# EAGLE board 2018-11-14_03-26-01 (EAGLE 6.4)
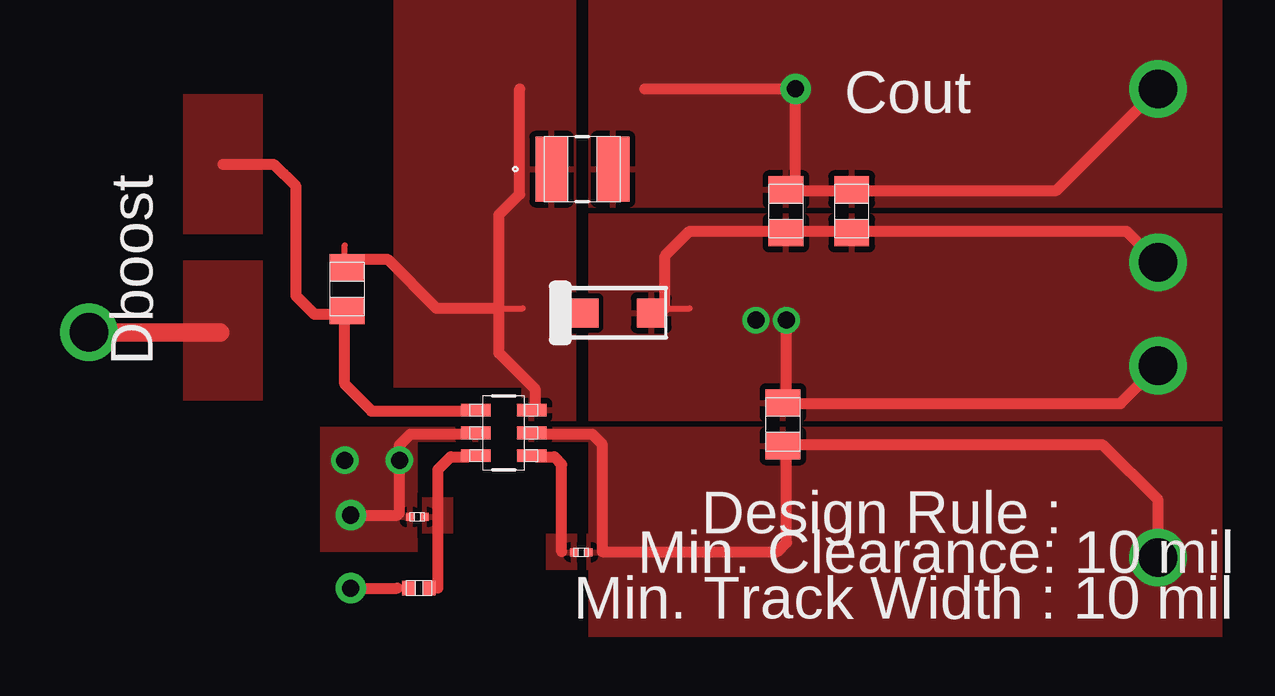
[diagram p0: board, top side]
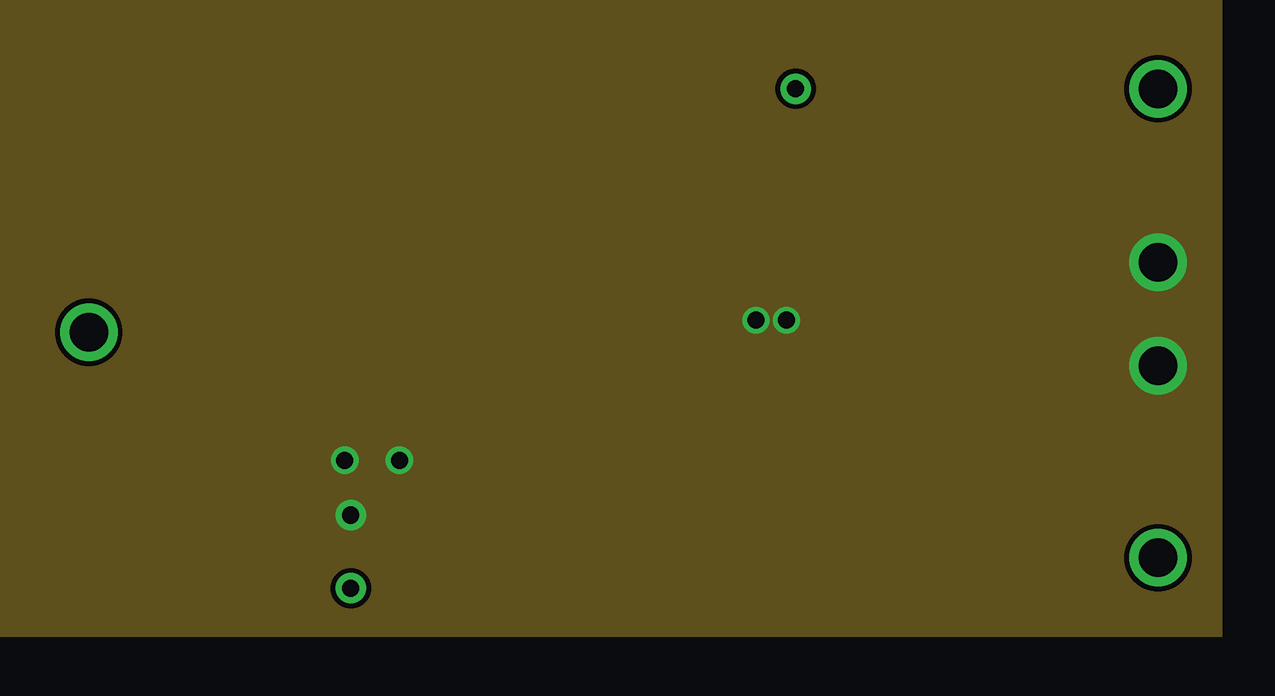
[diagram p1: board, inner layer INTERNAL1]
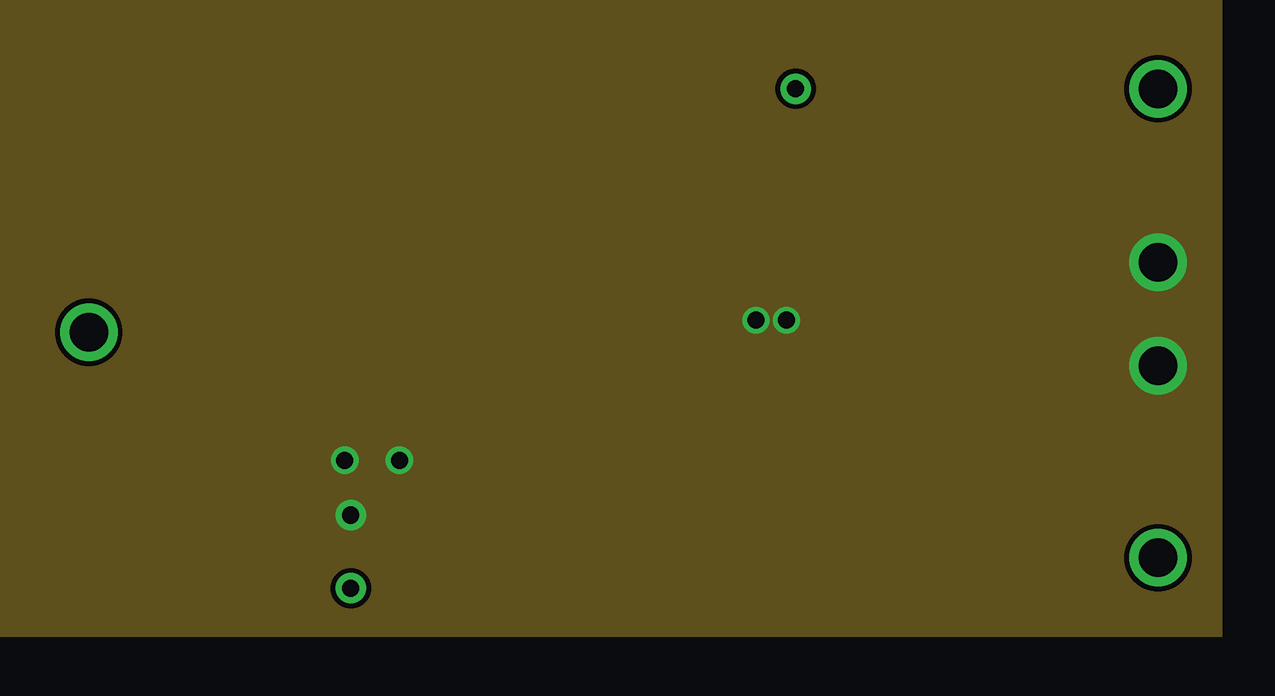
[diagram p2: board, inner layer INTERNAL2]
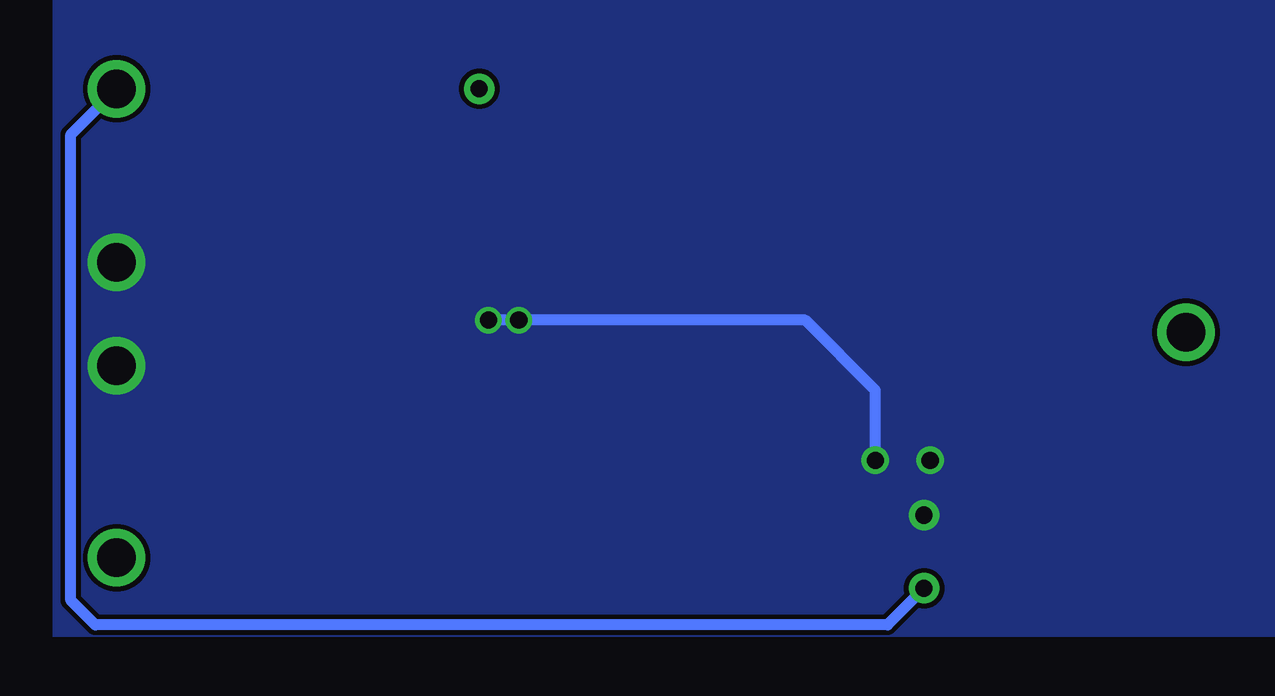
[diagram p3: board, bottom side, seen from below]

No outline drawn. Coordinates in mm, seen from the top.
Copper layers ((1*2)+(15*16)): TOP / INTERNAL1 / layer 15 / BOTTOM

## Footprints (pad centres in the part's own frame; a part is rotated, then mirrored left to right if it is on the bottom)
0805 = smd 1.118 x 1.448: 1 -0.902,0; 2 0.902,0
SOD-123F = smd 1.2 x 1.2: 1 -1.4,0; 2 1.4,0
TP-5012 = drill 0.813 round: 1 0,0
SRN3015 = smd 1.356 x 2.7: 1 -1.278,0; 2 1.278,0
0201 = smd 0.356 x 0.33: 1 -0.292,0; 2 0.292,0
0402 = smd 0.559 x 0.61: 1 -0.419,0; 2 0.419,0
MK06A = smd 1.219 x 0.533: 1 -1.168,0.95; 2 -1.168,0; 3 -1.168,-0.95; 4 1.168,-0.95; 5 1.168,0; 6 1.168,0.95

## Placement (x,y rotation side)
Cb  [0805]  40.49,40.41 90 top
Cin  [0805]  58.65,34.77 90 top
Cout_1  [0805]  58.78,43.66 270 top
Cout_2  [0805]  61.52,43.66 270 top
D1  [SOD-123F]  51.77,39.42 0 top
GND  [TP-5012]  74.3,37.19 90 top
GND1  [TP-5012]  74.3,41.48 90 top
L1  [SRN3015]  50.29,45.42 0 top
Renable  [0201]  50.24,29.44 0 top
Rfb1  [0201]  43.41,30.91 180 top
Rfb2  [0402]  43.48,27.94 0 top
U1  [MK06A]  47.02,34.42 0 top
Vin  [TP-5012]  74.3,29.18 90 top
Vout  [TP-5012]  74.3,48.72 90 top
Vsupply  [TP-5012]  29.67,38.58 90 top

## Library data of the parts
Cb = ultra-librarian; RefDes: Cb; Type: CGA4C2C0G1H103J060AA
Cin = ultra-librarian; RefDes: Cin; Type: C2012X5R1V226M125AC
Cout_1 Cout_2 = ultra-librarian
D1 = ultra-librarian; RefDes: D1; Type: MBR1020VL
GND = ultra-librarian; RefDes: GND; Type: TP-5012
GND1 = ultra-librarian; RefDes: GND1; Type: TP-5012
L1 = ultra-librarian; RefDes: L1; Type: SRN3015-6R8M
Renable = ultra-librarian; RefDes: Renable; Type: RC0201FR-0710KL
Rfb1 = ultra-librarian; RefDes: Rfb1; Type: RC0201FR-0710KL
Rfb2 = ultra-librarian; RefDes: Rfb2; Type: CRCW040234K0FKED
U1 = ultra-librarian; RefDes: U1; Type: LM2736XMK/NOPB
Vin = ultra-librarian; RefDes: Vin; Type: TP-5012
Vout = ultra-librarian; RefDes: Vout; Type: TP-5012
Vsupply = ultra-librarian; RefDes: Vsupply; Type: TP-5012

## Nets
0: Cin.2 Cout_1.2 Cout_2.2 D1.2 GND1.1 GND.1 Rfb1.2 U1.2
1: Cin.1 Renable.2 U1.5 Vin.1
2: Cb.1 U1.1
4: Rfb1.1 Rfb2.2 U1.3
5: Cout_1.1 Cout_2.1 L1.2 Rfb2.1 Vout.1
6: Cb.2 D1.1 L1.1 U1.6
7: Renable.1 U1.4
15: Vsupply.1

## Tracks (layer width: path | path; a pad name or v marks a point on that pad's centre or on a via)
0  (via drill 0.71 pad 1.02, 0.71 pad 1.14, 0.71 pad 1.27, 1.6 pad 2.21)
  TOP 0.254: 52.73,39.61 54.76,39.61
  TOP 0.457: v58.8,39.12 58.8,35.64 72.72,35.64 v74.3,37.21 | v74.3,41.53 72.97,42.82 59.18,42.82 54.76,42.82 53.75,41.81 53.75,39.62 | 42.67,31.06 v42.67,33.27 42.67,33.91 43.13,34.37 45.54,34.37 | v40.64,30.99 42.57,30.99
  BOTTOM 0.457: v42.67,33.27 42.67,35.05 42.67,36.2 45.59,39.12 v57.53,39.12 v58.8,39.12
  other vias: 40.39,33.27
  pour TOP (rank 6): 39.37,34.67 39.37,29.46 43.43,29.46 43.43,34.04 46.35,34.04 46.35,34.67
  pour TOP: 76.96,43.56 76.96,34.92 50.55,34.92 50.55,43.56
  pour BOTTOM (rank 6): 76.96,25.91 76.96,54.86 25.91,54.86 25.91,25.91
  pour INTERNAL2 (rank 5): 76.96,54.86 76.96,25.91 25.91,25.91 25.91,54.86
  pour INTERNAL1 (rank 5): 76.96,54.86 76.96,25.91 25.91,25.91 25.91,54.86
1  (via drill 1.6 pad 2.21)
  TOP 0.457: v74.3,29.21 74.3,31.62 71.96,33.93 58.8,33.93 58.8,29.84 58.42,29.46 51.13,29.46 51.13,33.93 50.7,34.37 48.34,34.37
  pour TOP (rank 2): 50.47,28.7 50.47,30.2 51.77,30.2 51.77,28.7
  pour TOP (rank 4): 76.96,34.67 76.96,25.91 50.55,25.91 50.55,34.04 47.75,34.04 47.75,34.67
2
  TOP 0.254: 40.39,38.79 40.39,39.95
  TOP 0.457: 45.54,35.33 41.5,35.33 40.39,36.45 40.39,39.37 39.12,39.37 38.35,40.13 38.35,44.7 37.41,45.62 | 35.31,45.62 37.41,45.62 | 37.41,45.62 37.85,45.21
  pour TOP (rank 2): 33.66,42.7 33.66,48.54 36.96,48.54 36.96,42.7
4
  TOP 0.457: 44.27,27.94 44.27,30.99 44.27,32.89 44.81,33.43 45.54,33.43
  pour TOP: 43.61,30.23 43.61,31.72 44.91,31.72 44.91,30.23
5  (via drill 0.71 pad 1.27, 1.6 pad 2.21)
  TOP 0.457: v74.3,48.77 70.05,44.53 59.18,44.53 v59.18,48.77 52.88,48.77 | v40.64,27.94 42.57,27.94
  BOTTOM 0.457: v74.3,48.77 76.2,46.86 76.2,27.43 75.18,26.42 42.16,26.42 v40.64,27.94
  pour TOP (rank 4): 76.96,54.86 76.96,43.81 50.55,43.81 50.55,54.86
6
  TOP 0.254: 40.39,41.07 40.39,42.24 | 45.77,39.61 47.8,39.61
  TOP 0.457: 40.39,41.66 42.16,41.66 44.2,39.62 46.81,39.62 | 46.81,39.62 46.81,37.74 48.34,36.22 48.34,35.33 | 46.81,39.62 46.81,43.51 47.68,44.37 47.68,48.77
  pour TOP (rank 3): 47.75,34.92 50.04,34.92 50.04,54.86 42.42,54.86 42.42,36.32 47.75,36.32
7
  TOP 0.457: 49.43,29.46 49.43,33.1 49.12,33.43 48.34,33.43
  pour TOP: 48.77,28.7 48.77,30.2 50.06,30.2 50.06,28.7
15  (via drill 1.6 pad 2.21)
  TOP 0.762: v29.72,38.61 35.2,38.61
  pour TOP (rank 3): 33.66,35.76 33.66,41.61 36.96,41.61 36.96,35.76

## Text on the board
ASSYNOTES: Cout | Dboost | Design Rule : | Min. Clearance: 10 mil | Min. Track Width : 10 mil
